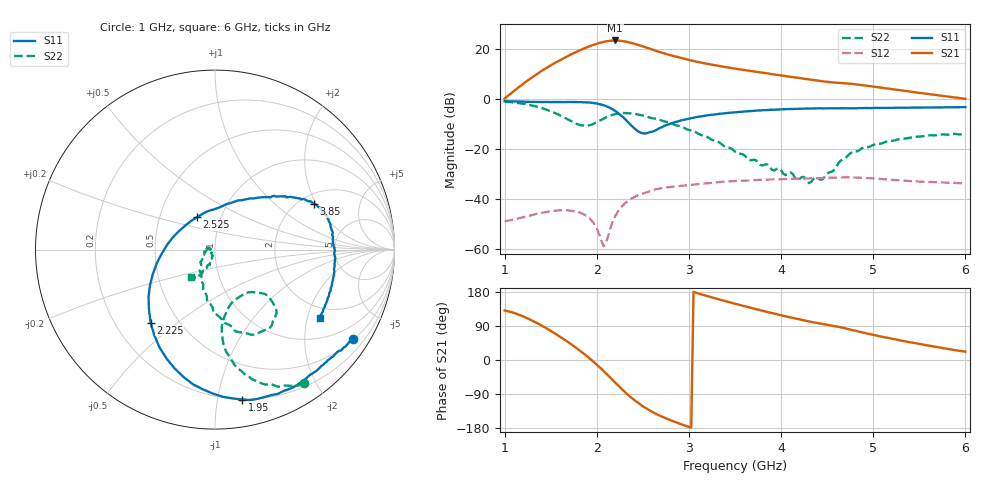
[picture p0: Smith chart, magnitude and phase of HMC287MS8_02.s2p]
!Hittite Microwave Corporation
!12 Elizabeth Drive
!Chelmsford, MA 01824
!Tel: 978-250-3343
!Fax: 978-250-3373
!Device: HMC287MS8, 2.3-2.5 GHz LNA with AGC in 8-lead Grounded Base surface Mount Plastic Package
!Misc: Vdd = +3V Idd = 9.6 mA Vctl = 0.2V.
# GHZ S DB R 50.0
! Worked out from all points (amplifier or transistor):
!   201 points, 1 GHz to 6 GHz, reference 50 ohm
!   highest |S21| = 23.6 dB at 2.2 GHz (marker M1)
!   |S21| within 3 dB of that: 1.876 GHz to 2.55 GHz (674.3 MHz wide, 30.5 % of centre)
!   unconditionally stable (mu >= 1): start of sweep to end of sweep
!   at 1.825 GHz: K = 2.33, MAG = 26.2 dB, |S12| = -45.5 dB
!   at 3.5 GHz: K = 3.68, MAG = 14.0 dB, |S12| = -32.8 dB
!   at 6 GHz: K = 11.82, MAG = 3.2 dB, |S12| = -33.7 dB
!   S11 on the Smith chart (normalised r, x): 1 GHz: 0.52, -3.31; 1.95 GHz: 0.20, -1.18; 2.225 GHz: 0.35, -0.40; 2.525 GHz: 0.77, +0.29; 3.85 GHz: 2.38, +1.91; 6 GHz: 1.63, -2.40
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1  -0.74 -32.9  0.22 130.8  -48.90 76.9  -0.97 -56.2
1.275  -1.03 -40.4  8.17 106.8  -46.64 75.6  -2.34 -72.9
1.475  -1.10 -46.7  13.03 80.7  -45.04 68.2  -4.44 -82.4
1.7  -1.10 -57.2  17.60 45.4  -44.59 51.3  -8.31 -82.5
1.85  -1.21 -68.5  20.16 18.5  -45.95 33.4  -10.51 -65.0
1.95  -1.42 -79.7  21.67 -1.4  -48.84 13.9  -10.09 -49.0
2.025  -1.91 -90.8  22.57 -17.9  -54.02 -12.7  -8.68 -41.9
2.075  -2.38 -99.3  23.03 -29.3  -58.89 -69.8  -7.79 -41.6
2.125  -3.11 -108.8  23.35 -41.2  -54.49 -142.5  -6.83 -43.3
2.2  -4.67 -125.4  23.58 -59.6  -46.88 -178.6  -5.95 -48.3
2.225  -5.31 -131.4  23.55 -65.8  -45.24 174.3  -5.80 -50.9
2.3  -7.70 -151.4  23.22 -83.2  -41.93 156.3  -5.52 -57.3
2.35  -9.56 -166.9  22.83 -94.2  -40.45 146.9  -5.62 -63.2
2.425  -12.20 164.2  22.06 -109.0  -38.84 135.2  -5.95 -68.4
2.525  -13.72 119.3  20.88 -125.8  -37.54 123.1  -6.70 -76.5
2.675  -11.68 76.1  19.02 -145.7  -35.84 108.7  -8.13 -84.3
3  -7.80 45.7  15.77 -176.6  -34.37 87.8  -12.31 -104.5
3.5  -5.22 31.4  12.29 148.7  -32.78 67.6  -20.99 -142.5
3.85  -4.33 24.7  10.38 126.9  -32.22 56.6  -26.12 179.3
4.35  -3.70 14.3  7.74 99.5  -31.67 44.1  -31.97 -164.3
5.175  -3.46 -8.8  4.24 57.5  -32.23 22.0  -16.74 -118.2
6  -3.14 -32.9  0.22 22.0  -33.73 15.9  -13.76 -131.0
